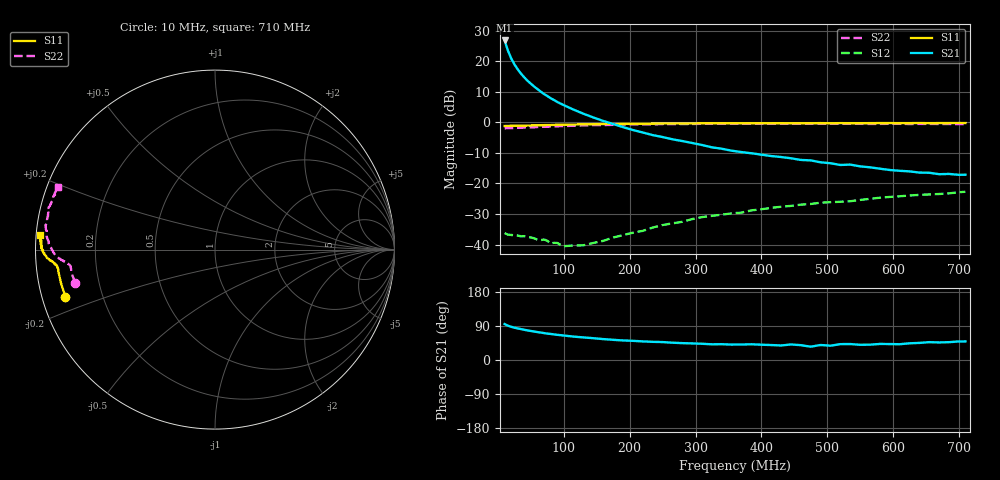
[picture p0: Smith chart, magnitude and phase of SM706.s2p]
!  POLYFET RF DEVICES
!  S PARAMETERS FOR
!  SM706
!  VDS=28, IDQ=800MA
! Date: Thu May 11 10:14:10 2000
# MHZ  S  MA  R  50.0000
! SCATTERING PARAMETERS :
! Freq=MHz Mag[s11] Ang[s11] Mag[s21] Ang[s21] Mag[s12] Ang[s12] Mag[s22] Ang[s22]
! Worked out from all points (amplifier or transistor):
!   60 points, 10 MHz to 710 MHz, reference 50 ohm
!   highest |S21| = 26.9 dB at 10 MHz (marker M1)
!   |S21| within 3 dB of that: start of sweep to 14.52 MHz
!   unconditionally stable (mu >= 1): 120.8 MHz to 251.9 MHz; 277.3 MHz to 287 MHz; 502.7 MHz to end of sweep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
!   at 60 MHz: K = 0.42, MSG = 24.7 dB, |S12| = -38.4 dB
!   at 280 MHz: K = 1.01, MAG = 12.6 dB, |S12| = -32.5 dB
!   at 710 MHz: K = 1.16, MAG = 0.4 dB, |S12| = -22.7 dB
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10  0.8736 -162.5  22 94.8  0.01535 4.6  0.8014 -166.7
15  0.8781 -167.6  15.01 90.6  0.01454 5.8  0.8082 -170.2
20  0.8794 -170.5  11.18 87.7  0.01435 5.0  0.809 -172.2
25  0.8811 -172.0  8.907 85.2  0.01416 1.3  0.8101 -173.4
30  0.8804 -173.0  7.371 83.4  0.01405 2.9  0.8152 -174.0
35  0.8844 -173.7  6.27 81.5  0.01361 0.7  0.8201 -174.3
40  0.885 -174.2  5.454 79.7  0.01371 1.3  0.8251 -174.6
45  0.8901 -174.5  4.791 78.1  0.01328 4.5  0.8285 -175.1
50  0.8913 -174.8  4.293 76.5  0.01308 1.2  0.8323 -175.1
60  0.8965 -175.1  3.506 73.6  0.01201 4.4  0.8426 -175.6
70  0.9033 -175.5  2.916 71.0  0.01207 8.2  0.8499 -175.9
80  0.9064 -175.8  2.494 68.7  0.01041 12.5  0.8587 -176.1
95  0.9145 -176.1  2.032 65.6  0.00988 17.5  0.8706 -176.7
115  0.9246 -176.5  1.615 61.7  0.00965 26.9  0.8833 -177.6
130  0.9297 -176.8  1.384 59.6  0.00972 42.0  0.8933 -178.3
160  0.9402 -177.5  1.055 55.2  0.0115 59.3  0.906 -179.8
190  0.9471 -178.1  0.8367 51.6  0.01428 69.2  0.9227 178.7
250  0.9579 -179.3  0.5767 47.3  0.02086 80.2  0.9376 176.1
370  0.9688 179.0  0.3267 40.9  0.03331 85.9  0.9484 170.5
490  0.9745 177.4  0.2223 39.6  0.04842 86.8  0.9568 165.9
595  0.9746 176.2  0.1663 42.1  0.06019 87.6  0.9485 161.9
710  0.9768 175.1  0.139 49.1  0.07321 90.1  0.9407 158.3
